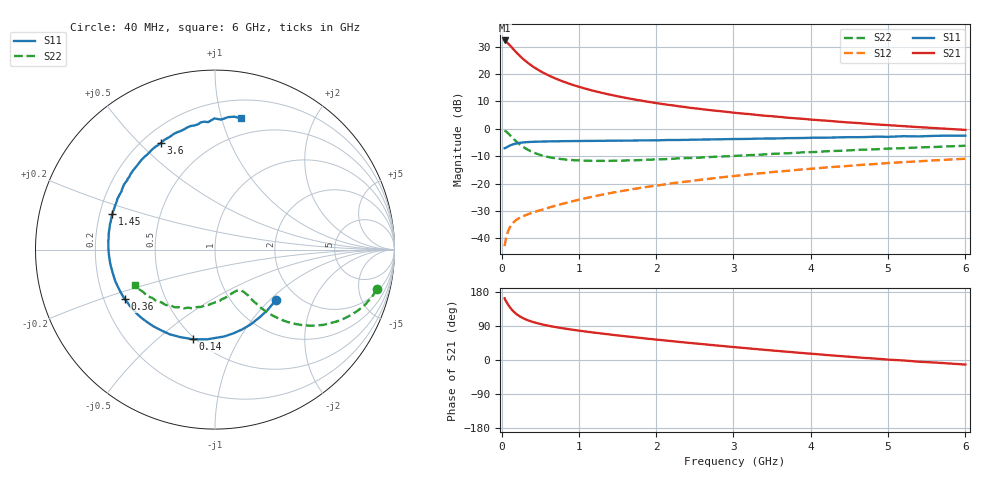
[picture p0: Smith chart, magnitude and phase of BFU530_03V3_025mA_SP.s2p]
! Filename:  P:\Prog\Test\Noise\ATS_data\Testdata_Net\03 Spar\BFU530_APG2013_40_A05_03p3V_025mA_SP_CM01_D.s2p
! Date/Time: Fri 26/Apr/2013 13:03:16
! BFU530_APG2013_40_A05_03p3V_1to25mA_SP_CM01_Bias8_R.s2p
! MDIF S-parameter v. bias file
! BFU530_APG2013_40_A05_03p3V_1to25mA_SP_CM01
! Date/time Wed Apr 24 18:17:07 2013
! VAR V_out= 3.3000
! VAR I_out= 25.0000
! VAR V_in= 0.8534
! VAR I_in= 0.2920
! Device data file deembeded for feedlines and parallel
! Original file: \03 Spar\BFU530_APG2013_40_A05_03p3V_025mA_SP_CM01_R.s2p
! Feed-files: PR047V01_250413_Feed1.s2p, PR047V01_250413_Feed2.s2p
! Parallel-file: PR047V01_250413_Par.s2p
# MHz S MA R 50
!  Freq-MHz  S11-mag  S11-arg  S21-mag  S21-arg  S12-mag  S12-arg  S22-mag  S22-arg
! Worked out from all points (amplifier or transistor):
!   98 points, 40 MHz to 6 GHz, reference 50 ohm
!   highest |S21| = 32.2 dB at 40 MHz (marker M1)
!   |S21| within 3 dB of that: start of sweep to 147.3 MHz
!   unconditionally stable (mu >= 1): 928.8 MHz to 3.142 GHz
!   at 300 MHz: K = 0.57, MSG = 28.3 dB, |S12| = -31.7 dB
!   at 1.6 GHz: K = 1.08, MAG = 15.2 dB, |S12| = -22.5 dB
!   at 6 GHz: K = 0.81, MSG = 5.3 dB, |S12| = -11.0 dB
!   S11 on the Smith chart (normalised r, x): 40 MHz: 1.56, -1.09; 140 MHz: 0.49, -0.66; 360 MHz: 0.29, -0.24; 1.45 GHz: 0.25, +0.16; 3.6 GHz: 0.27, +0.58; 6 GHz: 0.35, +1.16
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40  0.4407 -39.8  40.87 162.7  0.007185 77.7  0.929 -13.8
50  0.4461 -48.8  40.2 158.1  0.008739 74.5  0.9116 -17.1
80  0.4703 -71.7  36.62 147.8  0.01284 67.2  0.8394 -25.8
90  0.4786 -78.2  35.41 144.6  0.01403 65.0  0.8138 -28.3
120  0.5017 -95.0  31.96 136.1  0.01696 59.9  0.737 -34.6
140  0.5144 -103.9  29.73 131.4  0.01851 57.3  0.6897 -38.0
180  0.5352 -118.2  25.74 123.5  0.02108 53.6  0.6072 -43.0
200  0.5407 -123.8  24.01 120.3  0.02209 52.4  0.5721 -44.9
240  0.5532 -133.1  21.11 114.8  0.02383 51.0  0.5135 -47.7
300  0.5651 -143.5  17.74 108.4  0.02605 50.2  0.4479 -50.4
360  0.574 -151.2  15.2 103.5  0.02804 50.4  0.4011 -52.1
480  0.5824 -162.0  11.74 96.2  0.03194 52.2  0.3399 -53.7
650  0.5889 -172.4  8.849 88.7  0.03764 55.1  0.2961 -55.2
850  0.5942 179.2  6.838 82.0  0.04485 58.1  0.272 -57.2
1050  0.598 172.0  5.565 76.1  0.05248 60.0  0.2626 -60.3
1450  0.605 160.7  4.053 66.1  0.06866 61.8  0.2606 -67.5
2050  0.6168 147.3  2.867 52.9  0.09352 61.5  0.2767 -80.2
3100  0.65 125.7  1.904 32.4  0.1416 57.1  0.3247 -102.5
3600  0.6668 116.8  1.644 23.4  0.1665 53.6  0.3524 -112.1
4100  0.6871 107.8  1.433 15.0  0.1906 49.7  0.3787 -122.2
5200  0.7309 90.2  1.115 -1.2  0.2455 39.9  0.4412 -142.4
6000  0.7459 78.8  0.953 -12.1  0.283 31.7  0.489 -156.2
